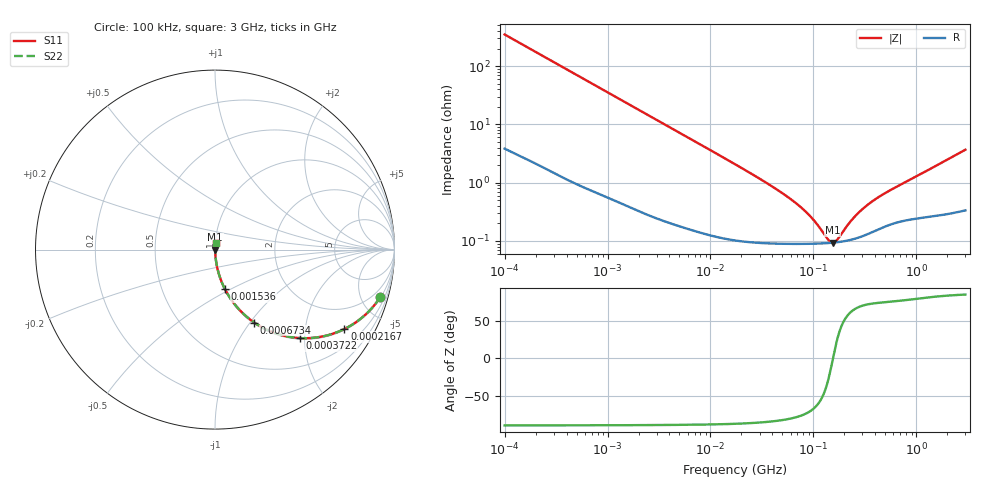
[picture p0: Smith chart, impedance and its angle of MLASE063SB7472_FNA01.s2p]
! MLASE063SB7472_FNA01  S-PARAMETER MODEL  ( Standard Model )
! Model Generated by TAIYO YUDEN Corporation (http://www.ty-top.com)
! Version 1.0
! TAIYO YUDEN Control No. 220601
! Copyright(c) 2009 TAIYO YUDEN CO.,LTD. All Rights Reserved.
! Product Description (link to TY-COMPAS)
! https://ds.yuden.co.jp/TYCOMPAS/or/detail?pn=MLASE063SB7472KFNA01&u=M
! Products Name : Multilayer Ceramic Capacitors
! Characteristics :
!  Capacitance : 4700 [pF] , Rated Voltage : 16 [V] , TCC : X7R
!  Case Size : 0.6 x 0.3 / 0.024 x 0.012 [mm/inch] , Thickness : 0.3 / 0.012 [mm/inch]
!  (Conditions: Temperature = 25 [degC] , DC Bias Voltage = 0 [V])
! External Node Assignments :
!  1  o---| |---o  2
! GND o---------o GND
! Frequency Range : 100kHz  -  3GHz  [ 401 STEP ]
# MHZ S RI R 50
! Freq[MHz].  S11 Real  S11 Imag  S21 Real  S21 Imag  S12 Real  S12 Imag  S22 Real  S22 Imag
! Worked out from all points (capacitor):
!   401 points, 100 kHz to 3 GHz, reference 50 ohm
!   read as one part in series: C = 4.56 nF near 105.3 kHz
!   lowest |Z| = 93.3 mohm at 154.9 MHz (marker M1)
!   series resonance near 155.2 MHz, so ESL is about 230 pH
!   S11 on the Smith chart (normalised r, x): 100 kHz: 1.08, -6.96; 216.7 kHz: 1.04, -3.23; 372.2 kHz: 1.02, -1.89; 673.4 kHz: 1.01, -1.05; 1.536 MHz: 1.01, -0.46; 3 GHz: 1.01, +0.07
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0.1  0.9213 -0.2638  0.0787 0.2638  0.0787 0.2638  0.9213 -0.2638
0.147195  0.8461 -0.3551  0.1539 0.3551  0.1539 0.3551  0.8461 -0.3551
0.216663  0.7205 -0.4427  0.2795 0.4427  0.2795 0.4427  0.7205 -0.4427
0.372249  0.4716 -0.4928  0.5284 0.4928  0.5284 0.4928  0.4716 -0.4928
0.562235  0.2848 -0.4445  0.7152 0.4445  0.7152 0.4445  0.2848 -0.4445
0.673391  0.2188 -0.4064  0.7812 0.4064  0.7812 0.4064  0.2188 -0.4064
0.991196  0.117 -0.3137  0.883 0.3137  0.883 0.3137  0.117 -0.3137
1.536162  0.0542 -0.218  0.9458 0.218  0.9458 0.218  0.0542 -0.218
3.161081  0.0149 -0.1112  0.9851 0.1112  0.9851 0.1112  0.0149 -0.1112
6.674626  0.0044 -0.0536  0.9956 0.0536  0.9956 0.0536  0.0044 -0.0536
17.7727  0.00141 -0.0201  0.9986 0.0201  0.9986 0.0201  0.00141 -0.0201
53.83243  0.000925 -0.00594  0.9991 0.00594  0.9991 0.00594  0.000925 -0.00594
75.25761  0.000901 -0.0037  0.9991 0.0037  0.9991 0.0037  0.000901 -0.0037
97.38194  0.000898 -0.00227  0.9991 0.00227  0.9991 0.00227  0.000898 -0.00227
139.694  0.000918 -0.000495  0.9991 0.000495  0.9991 0.000495  0.000918 -0.000495
154.8634  0.000932 -9.04e-06  0.9991 9.04e-06  0.9991 9.04e-06  0.000932 -9.04e-06
171.6802  0.00095 0.000477  0.999 -0.000477  0.999 -0.000477  0.00095 0.000477
227.9507  0.00104 0.00185  0.999 -0.00185  0.999 -0.00185  0.00104 0.00185
287.4592  0.00118 0.00306  0.9988 -0.00306  0.9988 -0.00306  0.00118 0.00306
381.6779  0.00146 0.00467  0.9985 -0.00467  0.9985 -0.00467  0.00146 0.00467
547.5153  0.00192 0.007  0.9981 -0.007  0.9981 -0.007  0.00192 0.007
3000  0.00465 0.0363  0.9953 -0.0363  0.9953 -0.0363  0.00465 0.0363
